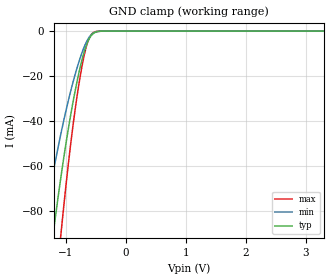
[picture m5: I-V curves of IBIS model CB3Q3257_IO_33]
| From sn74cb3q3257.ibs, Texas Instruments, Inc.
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[Model]   CB3Q3257_IO_33
Model_type  Terminator
| variable   typ   min   max
C_comp   7.02pF   5.12pF   11.50pF
| C_tri-state   7.02pF   5.12pF   11.50pF
[Temperature Range]   40   100   -40
| Ambient temperature   25   85   -40
[Voltage range]   3.3   3   3.6
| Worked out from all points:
|   GND clamp passes 1 mA (typ) near -0.54 V on its own axis
[GND Clamp]
| CB3Q3257_IO_33
|   Voltage   I(typ)   I(min)   I(max)
-5.5V     -1.394A    -1.081A    -1.727A
-1.38V    -127.2mA   -88.48mA   -178.7mA
-1.21V    -90.12mA   -62.84mA   -126.5mA
-1.19V    -86.02mA   -60.03mA   -120.7mA
-1.09V    -66.48mA   -46.67mA   -92.61mA
-1.07V    -62.78mA   -44.14mA   -87.25mA
-975mV    -46.24mA   -32.83mA   -63.2mA
-890mV    -33mA      -23.73mA   -44.03mA
-760mV    -15.99mA   -11.88mA   -20.09mA
-645mV    -5.457mA   -4.252mA   -5.685mA
-540mV    -1.025mA   -857.2uA   -630.8uA
3.3V      247.2pA    1.036nA    31.86pA
